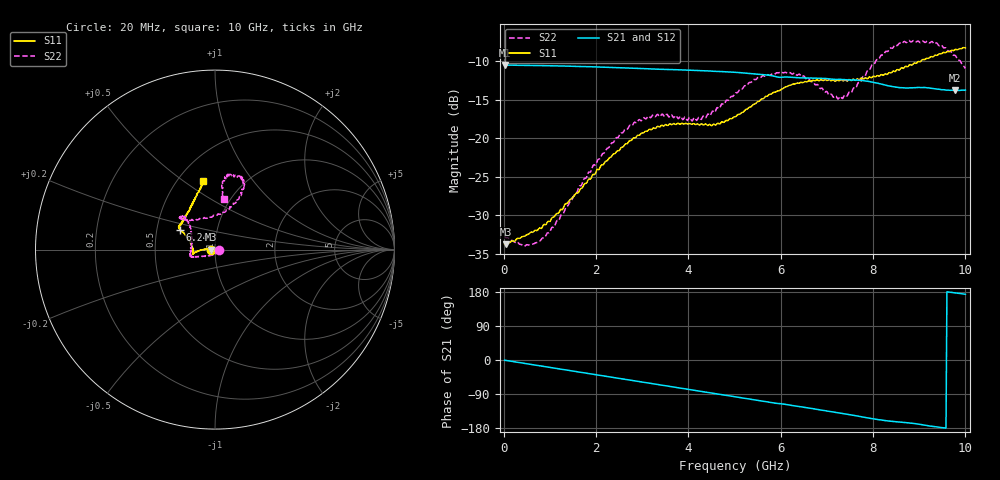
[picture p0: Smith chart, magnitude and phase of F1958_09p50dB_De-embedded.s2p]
! Integrated Device Technology
! Corporate Headquarters
! 6024 Silver Creek Valley Road
! San Jose, CA 95138  USA
! Phone:  1-408-284-8200
! Toll Free:  1-800-223-1366
! Webpage:  http://www.idt.com/
! Timing and RF Division
! 515 Groton Road, Suite 102
! Westford, MA 01886-6024
! Device:  F1958
! Description: 7-bit 0.25 dB Digital Step Attenuator
! Frequency:  0.001 -  6.000 GHz
! Package:  4x4 mm Thin QFN Plastic Package: 24 pin
! Ports:  2 RF, 12 DC
!  Pin  1  = D0
!  Pin  2  = VDD
!  Pin  3  = VMODE
!  Pin  4  = GND
!  Pin  5  = RF1  =  Port 1
!  Pin  6  = GND
!  Pin  7  = GND
!  Pin  8  = GND
!  Pin  9  = GND
!  Pin 10  = GND
!  Pin 11  = GND
!  Pin 12  = GND
!  Pin 13  = GND
!  Pin 14  = RF2  =  Port 2
!  Pin 15  = GND
!  Pin 16  = LE
!  Pin 17  = CLK
!  Pin 18  = DATA
!  Pin 19  = D6
!  Pin 20  = D5
!  Pin 21  = D4
!  Pin 22  = D3
!  Pin 23  = D2
!  Pin 24  = D1
! State:  38
! Atten State:  9.50 dB
! Voltage:  +3.30 Volts
! Current:  0.258 mA
! Data:  The device was measured on a F1958 evaluation board which has
!  individual transmission lines to the RF pins.  Data was collected
!  using a calibrated network analyzer.  The evaluation board was
!  de-embedded using Automatic Fixture Removal (AFR).
!  The reference plane is the edge of the package pin.
! Misc:
!  Action Tracker AT0419
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# GHz S dB R 50
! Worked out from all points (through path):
!   500 points, 20 MHz to 10 GHz, reference 50 ohm
!   highest |S21| = -10.45 dB at 20 MHz (marker M1); lowest = -13.8 dB at 9.78 GHz (marker M2)
!   group delay of S21, straight-line fit = 52.5 ps
!   lowest |S11| = -33.8 dB at 40 MHz (marker M3), VSWR 1.04, Z = 48 - j0.0726 ohm
!   |S11| at or under -10 dB: start of sweep to 9.028 GHz
!   |S22| runs from -34.0 to -7.3 dB; largest |S21 - S12| = 0.00083
!   S11 on the Smith chart (normalised r, x): 20 MHz: 0.96, -0.00; 6.24 GHz: 0.66, +0.15; 10 GHz: 0.66, +0.59
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0.02  -33.74 -177.8  -10.45 -0.5  -10.45 -0.5  -32.72 -5.5
0.04  -33.79 -177.9  -10.46 -0.9  -10.46 -0.9  -32.89 -8.4
0.44  -32.73 174.8  -10.52 -8.7  -10.52 -8.7  -34.02 -36.5
0.76  -31.74 174.6  -10.54 -14.9  -10.54 -14.9  -33.42 -65.8
1.1  -30.18 176.0  -10.57 -21.5  -10.57 -21.5  -31.48 -98.7
1.7  -26.47 178.6  -10.66 -33.0  -10.66 -33.0  -25.89 -138.0
2.58  -21.14 -175.2  -10.84 -50.0  -10.82 -50.1  -19.29 -158.5
2.92  -19.59 -172.8  -10.91 -56.6  -10.90 -56.7  -17.62 -162.1
3.36  -18.51 -170.1  -11.02 -65.0  -11.02 -65.2  -17.06 -164.7
4.24  -18.27 -173.9  -11.18 -81.9  -11.19 -81.9  -17.29 167.0
5.02  -17.20 166.3  -11.41 -97.0  -11.42 -97.0  -14.08 136.6
5.56  -15.02 154.7  -11.69 -107.4  -11.70 -107.4  -12.10 133.3
6.24  -13.03 150.2  -12.06 -119.9  -12.08 -119.8  -11.63 138.0
6.68  -12.50 148.0  -12.17 -128.0  -12.19 -128.0  -12.61 133.7
7.1  -12.51 144.1  -12.30 -136.8  -12.31 -136.7  -14.28 116.2
7.36  -12.53 141.7  -12.36 -141.7  -12.37 -141.6  -14.62 93.5
7.9  -12.13 131.4  -12.59 -153.0  -12.59 -153.1  -11.14 68.5
8.34  -11.49 121.9  -13.18 -161.0  -13.18 -161.1  -8.56 64.8
8.74  -10.71 114.6  -13.45 -165.6  -13.46 -165.5  -7.49 68.9
9.24  -9.41 105.4  -13.49 -174.4  -13.49 -174.5  -7.55 78.7
9.78  -8.44 100.8  -13.78 177.2  -13.81 177.3  -9.22 83.0
10  -8.24 100.3  -13.72 173.5  -13.75 173.6  -10.91 80.0
